FUNCTION "Gest Interfaccia" : VOID
TITLE =Gestione Interfaccia con altri quadri
AUTHOR : MassimoZ
FAMILY : NovaSrl
VERSION : 0.1

BEGIN
NETWORK
TITLE ======== Interfaccia Quadro Linea =======

NETWORK
TITLE =Posa Coperchi in Manuale
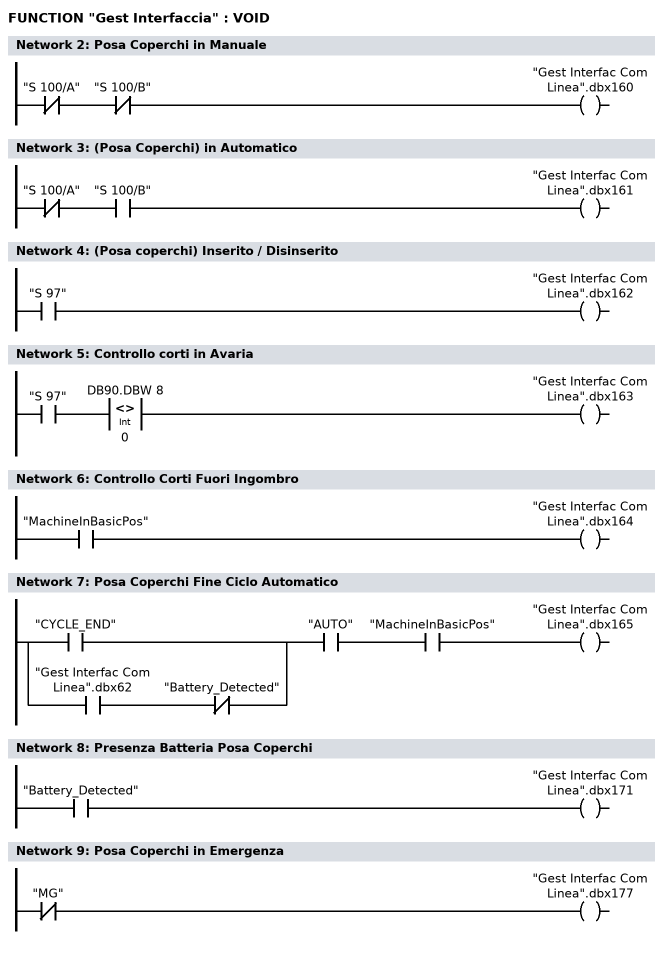
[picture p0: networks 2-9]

      UN    "S 100/A";
      UN    "S 100/B";
      =     "Gest Interfac Com Linea".dbx160;
NETWORK
TITLE =(Posa Coperchi) in Automatico

      UN    "S 100/A";
      U     "S 100/B";
      =     "Gest Interfac Com Linea".dbx161;
NETWORK
TITLE =(Posa coperchi) Inserito / Disinserito

      U     "S 97";
      =     "Gest Interfac Com Linea".dbx162;
NETWORK
TITLE =Controllo corti in Avaria

      U     "S 97";
      U(    ;
      L     DB90.DBW    8;
      L     0;
      <>I   ;
      )     ;
      =     "Gest Interfac Com Linea".dbx163;
NETWORK
TITLE =Controllo Corti Fuori Ingombro

      U     "MachineInBasicPos";
      =     "Gest Interfac Com Linea".dbx164;
NETWORK
TITLE =Posa Coperchi Fine Ciclo Automatico

      U(    ;
      O     "CYCLE_END";
      O     ;
      U     "Gest Interfac Com Linea".dbx62;
      UN    "Battery_Detected";
      )     ;
      U     "AUTO";
      U     "MachineInBasicPos";
      =     "Gest Interfac Com Linea".dbx165;
NETWORK
TITLE =Presenza Batteria Posa Coperchi

      U     "Battery_Detected";
      =     "Gest Interfac Com Linea".dbx171;
NETWORK
TITLE =Posa Coperchi in Emergenza

      UN    "MG";
      =     "Gest Interfac Com Linea".dbx177;
END_FUNCTION

